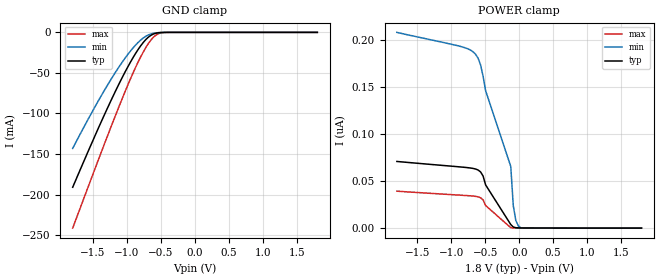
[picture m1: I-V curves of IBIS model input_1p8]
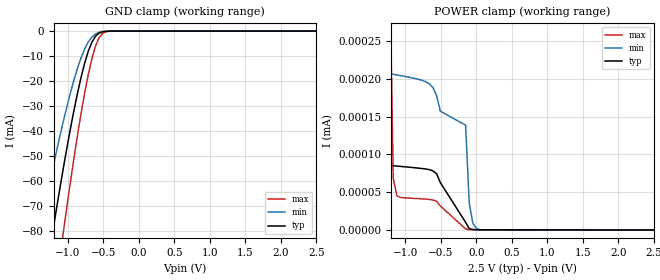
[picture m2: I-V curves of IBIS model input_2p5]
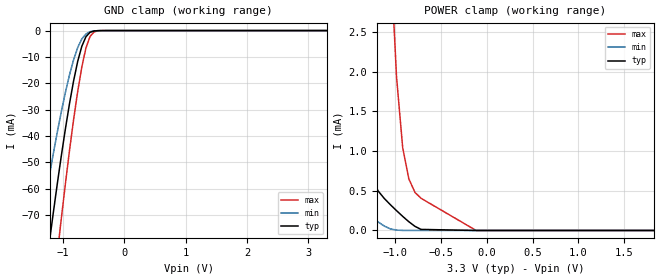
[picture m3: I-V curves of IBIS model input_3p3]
|Texas Instruments Incorporated
| 8-Bit Dual-Supply Bus Transceiver With Configurable Voltage Translation and
| 3-State Outputs
[IBIS Ver]   4.1
[File name]   txv0106.ibs
[Date]   12/05/2023
[File Rev]   1.0
[Source]
| Texas Instruments Incorporated.
| Analog-eLab Design Center, HPA
| 12500 TI Blvd
| Dallas, TX -75243
[Notes]
| Rev 1.0: 12/05/2023
| - Initial release
[Disclaimer]
| This model is designed as an aid for customers of Texas Instruments.
| TI and its licensors and suppliers make no warranties, either expressed
| or implied, with respect to this  model, including the warranties of
| merchantability or fitness for a particular purpose. The model is
| provided solely on an "as is" basis. The entire risk as to its quality
| and performance is with the customer.
[Copyright]
(C) Copyright 2017 Texas Instruments Incorporated.All rights reserved.
|   TXV0106BQB
| Marketing part#   Digital Voltage Range   Package-type   #pins
| TXV0106BQB   1.8V-3.6V   WQFN   16
[Component]   TXV0106BQB
[Manufacturer]  TI
[Package]   |16 WQFN - BQB package
|   typ   min   max
R_pkg   0.05   0.04   0.06
L_pkg   1.0nH   0.8nH   1.2nH
C_pkg   0.2pF   0.16pF   0.24pF
[Pin]  signal_name   model_name   R_pin   L_pin   C_pin
1   VCCA   POWER   NA   NA   NA
2   A1   input   NA   NA   NA
3   A2   input   NA   NA   NA
4   A3   input   NA   NA   NA
5   A4   input   NA   NA   NA
6   A5   input   NA   NA   NA
7   A6   input   NA   NA   NA
8   GND   GND   NA   NA   NA
9   NOE   input   NA   NA   NA
10   B6   output   NA   NA   NA
11   B5   output   NA   NA   NA
12   B4   output   NA   NA   NA
13   B3   output   NA   NA   NA
14   B4   output   NA   NA   NA
15   B1   output   NA   NA   NA
16   VCCB   POWER   NA   NA   NA
|   TXV0106BQB
| Marketing part#   Digital Voltage Range   Package-type   #pins
| TXV0106BQB   1.8V-3.6V   WQFN   16
[Model Selector] input
input_1p8   1.8V   digital Input
input_2p5   2.5V   digital Input
input_3p3   3.3V   digital Input
[Model Selector] output
output_1p8   1.8V   digital Output
output_2p5   2.5V   digital Output
output_3p3   3.3V   digital Output
| Models and submodels in the file (6): input_1p8 (Input), input_2p5 (Input), input_3p3 (Input), output_1p8 (I/O), output_2p5 (I/O), output_3p3 (I/O)
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|   input_1p8 Model
[Model]   input_1p8
Model_type   Input
Vinl =  0.540V
Vinh =  1.260V
|   typ   min   max
C_comp   1.986pF   1.912pF   2.111pF
| Where Nom  PVT is Nominal Process, 1.8V,  27C
|   Fast PVT is Strong Process,  1.95V, -40C
|   Slow PVT is Weak Process,   1.65V, 125C
[Voltage Range]   1.8   1.65   1.95
|Junction Temperature
[Temperature Range]   27   125   -40
[Power Clamp Reference]   1.8   1.65   1.95
[GND Clamp Reference]   0   0   0
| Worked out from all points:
|   GND clamp passes 1 mA (typ) near -0.57 V on its own axis
[GND Clamp]
|Voltage   I(typ)   I(min)   I(max)
-1.8V     -191mA     -143.1mA   -241.4mA
-1.578V   -147.8mA   -107.9mA   -191.8mA
-1.356V   -105.8mA   -74.75mA   -142.6mA
-1.171V   -72.59mA   -49.3mA    -102.6mA
-986mV    -42.13mA   -26.9mA    -64.4mA
-875mV    -26.05mA   -15.67mA   -43.28mA
-764mV    -12.71mA   -7.063mA   -24.62mA
-653mV    -3.853mA   -2.076mA   -9.887mA
-579mV    -1.121mA   -675.7uA   -3.576mA
-505mV    -223.2uA   -170.7uA   -768.7uA
-394mV    -11.53uA   -14.74uA   -30.66uA
1.8V      0A         0A         0A
[POWER Clamp]
|Voltage   I(typ)   I(min)   I(max)
-1.8V     70.75nA    207.7nA    39.26nA
-790mV    64.4nA     191.2nA    34.62nA
-679mV    63.35nA    187.1nA    34.01nA
-605mV    61.67nA    180.3nA    33.2nA
-568mV    59.62nA    173.1nA    32.21nA
-531mV    55.25nA    161nA      29.88nA
-494mV    45.84nA    145.8nA    23.95nA
-124mV    3.805nA    65.43nA    485.7pA
-87mV     1.147nA    23.84nA    235.2pA
-50mV     439pA      8.249nA    184.2pA
-13mV     246.6pA    2.405nA    165pA
1.8V      0A         0A         0A
|   input_2p5 Model
[Model]   input_2p5
Model_type   Input
Vinl = 0.75
Vinh = 1.75
|   typ   min   max
C_comp   1.985pF   1.882pF   2.077pF
| Where Nom  PVT is Nominal Process, 2.5V, 27C
|   Fast PVT is Strong Process,  2.70V, -40C
|   Slow PVT is Weak Process,   2.25, 125C
[Voltage Range]   2.5   2.25   2.75
|Junction Temperature
[Temperature Range]   27   150   -40
[Power Clamp Reference]   2.50   2.25   2.70
[GND Clamp Reference]   0   0   0
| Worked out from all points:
|   GND clamp passes 1 mA (typ) near -0.57 V on its own axis
|   POWER clamp passes 1 mA (typ) near -2.11 V on its own axis
[GND Clamp]
|Voltage   I(typ)   I(min)   I(max)
-2.092V   -248.6mA   -191.1mA   -306.3mA
-1.429V   -119.5mA   -85.39mA   -158.7mA
-1.378V   -109.9mA   -77.92mA   -147.5mA
-1.225V   -82.07mA   -56.47mA   -114.1mA
-1.174V   -73.11mA   -49.69mA   -103.2mA
-1.072V   -55.84mA   -36.85mA   -81.8mA
-817mV    -18.65mA   -10.78mA   -33.14mA
-715mV    -8.118mA   -4.382mA   -17.51mA
-613mV    -2.08mA    -1.169mA   -6.039mA
-511mV    -257.4uA   -192.5uA   -888.4uA
-409mV    -17.82uA   -20.92uA   -50.46uA
2.5V      0A         0A         0A
[POWER_clamp]
|Voltage   I(typ)   I(min)   I(max)
-2.5V     9.06mA     1.505mA    24mA
-1.631V   89.37uA    412nA      361.9uA
-1.427V   634.6nA    210.9nA    115.9uA
-1.325V   97.17nA    208.6nA    22.38uA
-1.223V   85.67nA    206.8nA    356.7nA
-1.172V   85.03nA    205.9nA    68.45nA
-1.121V   84.55nA    205.1nA    45.15nA
-560mV    74.27nA    177.6nA    37.88nA
-152mV    10.06nA    138.6nA    1.335nA
-101mV    1.901nA    35.68nA    364.7pA
1mV       333.1pA    1.981nA    228.7pA
2.5V      0A         0A         0A
|   input_3p3 Model
[Model]   input_3p3
Model_type   Input
Vinl =  0.500V
Vinh =  2.310V
|   typ   min   max
C_comp   1.956pF   1.864pF   1.998pF
| Where Nom  PVT is Nominal Process, 3.3V, 27C
|   Fast PVT is Strong Process,  3.6V, -40C
|   Slow PVT is Weak Process,   3.0V, 130C
[Voltage Range]   3.3   3   3.6
|Junction Temperature
[Temperature Range]   27   125   -40
[Power Clamp Reference]   3.3   3   3.6
[GND Clamp Reference]   0   0   0
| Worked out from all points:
|   GND clamp passes 1 mA (typ) near -0.57 V on its own axis
|   POWER clamp passes 1 mA (typ) near -1.32 V on its own axis
[GND Clamp]
|Voltage   I(typ)   I(min)   I(max)
-2.161V   -262.3mA   -202.7mA   -322.1mA
-1.357V   -106mA     -74.89mA   -142.8mA
-1.223V   -81.71mA   -56.2mA    -113.7mA
-1.156V   -69.99mA   -47.35mA   -99.38mA
-1.089V   -58.65mA   -38.91mA   -85.32mA
-1.022V   -47.76mA   -30.95mA   -71.6mA
-821mV    -19.13mA   -11.09mA   -33.81mA
-687mV    -5.965mA   -3.194mA   -13.85mA
-620mV    -2.337mA   -1.299mA   -6.642mA
-553mV    -661uA     -428.6uA   -2.22mA
-419mV    -23.68uA   -26.36uA   -69.53uA
3.3V      0A         0A         0A
[POWER_clamp]
|Voltage   I(typ)   I(min)   I(max)
-2.395V   12.55mA    3.763mA    27.8mA
-2.06V    10.25mA    2.495mA    24.28mA
-1.591V   5.721mA    630.5uA    16.83mA
-1.457V   3.172mA    377.4uA    13.63mA
-1.323V   1.023mA    231.1uA    10.42mA
-1.122V   403uA      55.42uA    5.418mA
-1.055V   324.2uA    19.6uA     3.488mA
-921mV    178uA      813.6nA    1.046mA
-854mV    110.8uA    273.9nA    652.3uA
-720mV    13.42uA    181.7nA    405.2uA
-117mV    3.335nA    55.92nA    606.8pA
1.826V    63.87pA    0A         113.5pA
